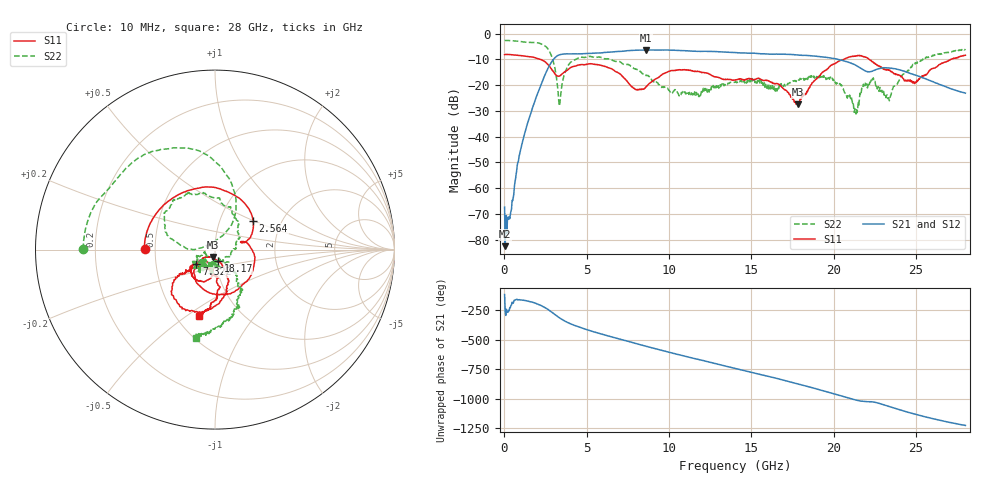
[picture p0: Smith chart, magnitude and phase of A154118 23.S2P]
!  2-Port S-parameters saved by WinCal
! VAR MeasName=S-Parameters (CALIBRATED_DATA) read from VNA (N5230A)
! VAR MeasDate=2015-9-10 14:36:07
! VAR NAME=A154118 23
! VAR FILENAME=A154118 23.S2P
! VAR DATE=2015-9-10 14:36:07
! VAR PHYS_PORTS=1,2
# Hz S DB R 50
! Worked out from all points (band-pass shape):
!   801 points, 10 MHz to 28 GHz, reference 50 ohm
!   highest |S21| = -6.35 dB at 8.582 GHz (marker M1); lowest = -82.5 dB at 44.99 MHz (marker M2)
!   |S21| within 3 dB of the highest: 3.072 GHz to 19.66 GHz (16.59 GHz wide, 146 % of centre)
!   lowest |S11| = -27.5 dB at 17.82 GHz (marker M3), VSWR 1.09, Z = 48.6 - j3.93 ohm
!   |S11| at or under -10 dB: 2.189 GHz to 20.62 GHz (18.43 GHz wide, 162 % of centre); 22.16 GHz to 27.13 GHz (4.965 GHz wide, 20.1 % of centre)
!   |S22| runs from -31.2 to -2.7 dB; largest |S21 - S12| = 0.0078
!   S11 on the Smith chart (normalised r, x): 10 MHz: 0.44, +0.00; 2.564 GHz: 1.44, +0.50; 7.322 GHz: 0.80, -0.13; 18.17 GHz: 1.02, -0.13; 28 GHz: 0.65, -0.56
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1e7  -8.19 179.6  -67.37 -114.9  -67.37 -138.9  -2.67 179.8
4.49875e7  -8.13 178.0  -82.52 101.8  -82.27 47.4  -2.69 178.9
2.899e8  -8.12 165.9  -71.09 108.8  -68.92 99.2  -2.71 172.9
1.26955e9  -8.76 118.8  -37.78 -165.9  -37.81 -165.4  -3.34 149.1
2.564088e9  -11.48 37.3  -14.60 126.0  -14.57 126.4  -5.35 96.7
3.333812e9  -16.49 16.8  -8.26 48.3  -8.23 48.3  -28.10 110.7
3.893612e9  -13.83 1.0  -7.88 4.4  -7.85 4.6  -12.14 166.2
4.698325e9  -12.01 -44.4  -7.85 -39.0  -7.82 -38.9  -9.16 142.3
7.322388e9  -17.58 -141.5  -6.77 -144.6  -6.72 -144.9  -12.09 75.0
8.581938e9  -20.79 -101.7  -6.35 167.1  -6.32 166.7  -16.23 28.8
9.351662e9  -17.08 -97.3  -6.45 139.1  -6.40 138.7  -19.74 2.7
1.1206e10  -14.14 -131.2  -6.75 73.4  -6.70 72.7  -23.64 -87.9
1.4005e10  -18.06 -137.0  -7.39 -21.2  -7.39 -21.7  -18.85 -120.9
1.781864e10  -27.46 -107.7  -8.30 -153.0  -8.29 -153.5  -18.43 -123.7
1.816851e10  -23.50 -76.3  -8.46 -165.2  -8.50 -165.6  -17.41 -119.7
1.869332e10  -19.13 -63.9  -8.66 174.7  -8.64 174.4  -16.29 -123.1
2.037272e10  -10.48 -85.3  -10.24 108.6  -10.10 107.8  -19.40 -160.9
2.131739e10  -8.80 -111.0  -12.21 71.0  -12.10 70.4  -30.46 -90.0
2.233202e10  -10.92 -143.1  -14.62 54.5  -14.61 53.5  -17.64 -97.4
2.334666e10  -14.24 -141.8  -13.34 16.0  -13.26 14.8  -25.11 -59.6
2.495609e10  -18.82 -105.4  -16.09 -50.0  -16.11 -51.0  -11.79 -56.1
2.8e10  -8.42 -103.2  -23.12 -145.6  -23.16 -146.7  -6.00 -102.1
